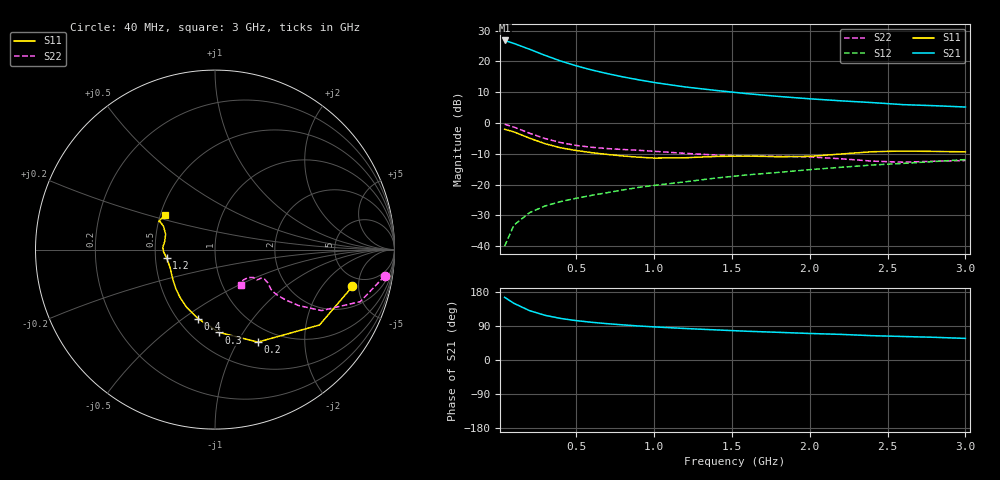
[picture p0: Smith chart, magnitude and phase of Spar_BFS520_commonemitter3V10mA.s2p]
! Filename:  BFS520C.S2P  Version:  4.0
! NXP part #: BFS520  Date: Jun 1994
! Bias condition: Vce=3V, Ic=10mA
#  MHz  S  MA  R  50
! Freq  S11  S21  S12  S22  !GUM [dB]
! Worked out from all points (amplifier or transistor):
!   21 points, 40 MHz to 3 GHz, reference 50 ohm
!   highest |S21| = 26.8 dB at 40 MHz (marker M1)
!   |S21| within 3 dB of that: start of sweep to 207.3 MHz
!   unconditionally stable (mu >= 1): 846.1 MHz to end of sweep
!   at 300 MHz: K = 0.63, MSG = 24.5 dB, |S12| = -26.9 dB
!   at 1 GHz: K = 1.05, MAG = 15.3 dB, |S12| = -20.3 dB
!   at 3 GHz: K = 1.06, MAG = 7.1 dB, |S12| = -11.9 dB
!   lowest NFmin = 1.10 dB at 500 MHz
!   S11 on the Smith chart (normalised r, x): 40 MHz: 3.83, -4.24; 200 MHz: 0.80, -1.22; 300 MHz: 0.67, -0.79; 400 MHz: 0.63, -0.57; 1.2 GHz: 0.57, -0.06; 3 GHz: 0.53, +0.23
40  0.793 -15.0  21.96 165.5  0.01 82.3  0.956 -8.9
100  0.718 -35.8  19.61 149.5  0.022 71.5  0.86 -19.7
200  0.568 -65.1  15.81 130.3  0.035 62.8  0.684 -29.8
300  0.462 -87.1  12.58 117.9  0.045 60.1  0.56 -33.8
400  0.396 -103.8  10.18 109.7  0.053 60.5  0.482 -35.5
500  0.358 -116.3  8.508 103.9  0.06 61.5  0.433 -36.1
600  0.33 -126.2  7.279 99.5  0.067 62.8  0.404 -36.0
700  0.309 -134.8  6.354 95.8  0.074 64.3  0.385 -35.5
800  0.292 -142.3  5.624 92.7  0.082 65.7  0.372 -34.5
900  0.279 -149.9  5.046 89.8  0.09 66.5  0.361 -33.4
1000  0.27 -157.1  4.562 87.4  0.097 67.4  0.348 -32.2
1200  0.273 -169.9  3.86 83.1  0.111 68.8  0.322 -30.8
1400  0.287 -177.7  3.383 79.4  0.128 70.1  0.302 -31.8
1600  0.291 177.4  2.999 75.8  0.144 70.2  0.292 -34.8
1800  0.284 171.2  2.706 73.0  0.158 71.0  0.288 -35.8
2000  0.288 162.7  2.476 70.0  0.175 71.0  0.282 -35.5
2200  0.314 155.8  2.297 67.6  0.191 71.4  0.263 -36.1
2400  0.342 153.1  2.15 64.2  0.208 71.2  0.241 -40.3
2600  0.351 153.3  1.991 62.0  0.221 70.6  0.231 -47.4
2800  0.346 151.1  1.914 59.9  0.237 70.8  0.24 -52.2
3000  0.341 145.4  1.821 57.0  0.255 70.4  0.246 -53.9
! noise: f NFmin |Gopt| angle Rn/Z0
500  1.1  0.716  32  0.19
900  1.25  0.318  59  0.16
2000  1.9  0.257  -171  0.15
